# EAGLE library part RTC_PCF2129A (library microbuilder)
PCF2120A - High Accuracy, Temp Compensated RTC with Integrated Crystal Digikey: 568-4960-5-ND
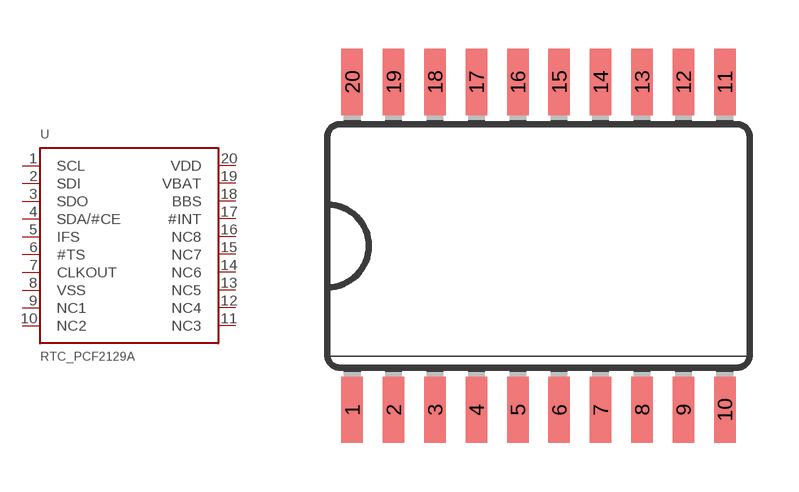
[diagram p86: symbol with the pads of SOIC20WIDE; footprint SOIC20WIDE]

Designator prefix U

## RTC_PCF2129A (PARTNO: PCF2129AT/1,512)  [SOIC20WIDE]
1  SCL
2  SDI
3  SDO
4  SDA/#CE
5  IFS
6  #TS
7  CLKOUT
8  VSS
9  NC1
10  NC2
11  NC3
12  NC4
13  NC5
14  NC6
15  NC7
16  NC8
17  #INT
18  BBS
19  VBAT
20  VDD

## Footprint SOIC20WIDE (pad centres in mm)
smd 0.66 x 2.032: 1 -5.715,-5.029; 2 -4.445,-5.029; 3 -3.175,-5.029; 4 -1.905,-5.029; 5 -0.635,-5.029; 6 0.635,-5.029; 7 1.905,-5.029; 8 3.175,-5.029; 9 4.445,-5.029; 10 5.715,-5.029; 11 5.715,5.029; 12 4.445,5.029; 13 3.175,5.029; 14 1.905,5.029; 15 0.635,5.029; 16 -0.635,5.029; 17 -1.905,5.029; 18 -3.175,5.029; 19 -4.445,5.029; 20 -5.715,5.029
